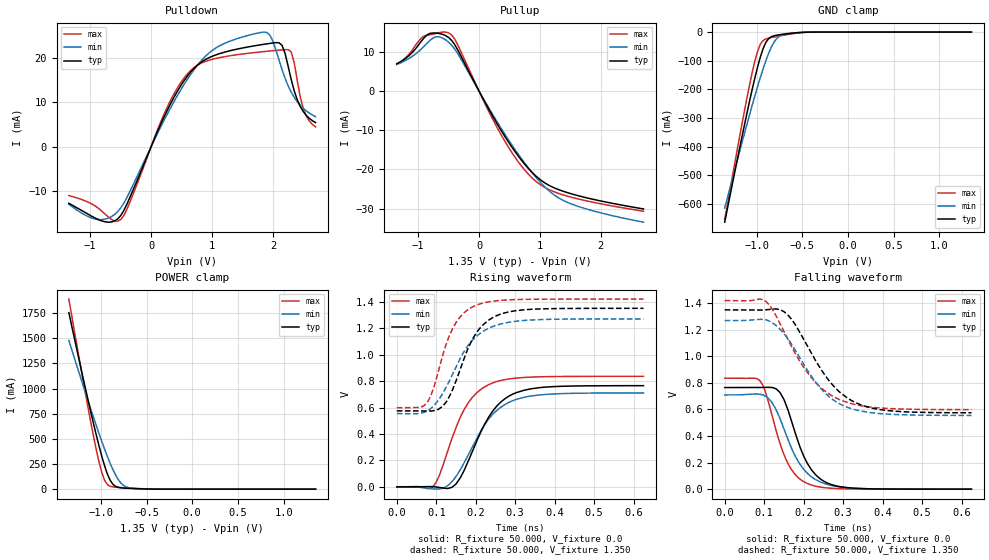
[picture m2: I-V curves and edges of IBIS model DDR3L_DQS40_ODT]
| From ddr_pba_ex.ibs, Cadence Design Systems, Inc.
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|   Model DDR3L_DQS40_ODT
[Model]   DDR3L_DQS40_ODT
Model_type I/O
Polarity   Non-Inverting
Enable   Active-High
Vinl   =   0.624V
Vinh   =   0.727V
C_comp   1.684pF   1.658pF   1.703pF
C_comp_pullup   0.506pF   0.522pF   0.489pF
C_comp_pulldown 1.177pF   1.136pF   1.213pF
[Model Spec]
Vinh   0.727V   NA   NA
Vinl   0.624V   NA   NA
Vmeas   0.675V   NA   NA
[Add Submodel]
|  Submodel_name   Mode
DDR3L_DQS_ODT60   Non-Driving
[Temperature Range]   27.000   0.125k   -40.000
[Voltage Range]   1.350V   1.270V   1.420V
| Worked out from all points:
|   slope of the pulldown table from 0 to 0.203 V, typ, clamps not added: 31.7 ohm
|   slope of the pullup table from 0 to 0.203 V, typ, clamps not added: 35 ohm
|   GND clamp passes 1 mA (typ) near -0.50 V on its own axis
|   POWER clamp passes 1 mA (typ) near -0.46 V on its own axis
|   rising waveform, R_fixture 50.000, V_fixture 0.0: 20-80 % time 78.8ps typ, 86.4ps min, 71.6ps max; typ from 0 V to 0.765 V
|   rising waveform, R_fixture 50.000, V_fixture 1.350: 20-80 % time 68.6ps typ, 82.9ps min, 58.3ps max; typ from 0.575 V to 1.35 V
|   falling waveform, R_fixture 50.000, V_fixture 0.0: 20-80 % time 59.7ps typ, 67.6ps min, 55.4ps max; typ from 0.765 V to 0 V
|   falling waveform, R_fixture 50.000, V_fixture 1.350: 20-80 % time 104ps typ, 102ps min, 106ps max; typ from 1.35 V to 0.575 V
[Pulldown]
|Voltage   I(typ)   I(min)   I(max)
-1.35V    -12.71mA   -12.95mA   -11mA
-850mV    -16.48mA   -16.4mA    -14.01mA
-500mV    -15.51mA   -13.79mA   -16.4mA
200mV     6.324mA    5.595mA    6.939mA
500mV     14.01mA    13.08mA    14.69mA
900mV     19.68mA    20.46mA    19.24mA
1.35V     21.77mA    24.03mA    20.58mA
1.95V     23.25mA    25.11mA    21.53mA
2.15V     22.81mA    17.35mA    21.79mA
2.3V      15.11mA    12.27mA    21.33mA
2.5V      7.867mA    8.611mA    8.524mA
2.7V      5.436mA    6.755mA    4.464mA
[Pullup]
|Voltage   I(typ)   I(min)   I(max)
-1.35V    6.994mA    6.778mA    6.785mA
-1.1V     9.771mA    8.81mA     10.37mA
-850mV    14.35mA    12.26mA    14.25mA
-700mV    14.79mA    13.87mA    14.72mA
-500mV    13.68mA    12.48mA    14.85mA
-350mV    10.51mA    9.572mA    11.81mA
400mV     -10.97mA   -10.4mA    -12.15mA
650mV     -16.69mA   -16.24mA   -18.16mA
900mV     -21.19mA   -21.37mA   -22.58mA
1.2V      -24.45mA   -26.1mA    -25.49mA
1.45V     -25.91mA   -28.39mA   -26.8mA
2.7V      -30.07mA   -33.45mA   -30.65mA
[GND_clamp]
|Voltage   I(typ)   I(min)   I(max)
-1.35V    -663.5mA   -614.2mA   -654.4mA
-1.17V    -379.6mA   -396.8mA   -336.4mA
-1.05V    -201.2mA   -256.6mA   -142.3mA
-990mV    -121.8mA   -190.1mA   -66.76mA
-960mV    -87.12mA   -158.5mA   -42.47mA
-930mV    -58.01mA   -128.3mA   -29.57mA
-870mV    -23.03mA   -74.64mA   -21.11mA
-810mV    -12.75mA   -34.94mA   -17.06mA
-750mV    -9.219mA   -14.09mA   -13.42mA
-690mV    -6.687mA   -6.669mA   -9.983mA
-420mV    -175.8uA   -266.9uA   -234.9uA
1.35V     1.781nA    307.1nA    267.4pA
[POWER_clamp]
|Voltage   I(typ)   I(min)   I(max)
-1.35V    1.755A     1.479A     1.89A
-1.17V    1.006A     962.6mA    958.1mA
-1.05V    538.4mA    632.4mA    392.2mA
-990mV    328mA      475.7mA    167mA
-960mV    234.7mA    400.6mA    90.32mA
-930mV    154.2mA    328.7mA    47.17mA
-900mV    91.53mA    260.8mA    29.3mA
-870mV    50.28mA    198.1mA    22.68mA
-780mV    13.3mA     60.49mA    15.94mA
-720mV    9.309mA    21.57mA    12.7mA
-660mV    6.902mA    8.818mA    9.643mA
1.35V     -4.773nA   -193.5nA   -1nA
[Ramp]
| variable   typ   min   max
dV/dt_r 0.459/79.862p   0.426/87.109p   0.502/73.280p
dV/dt_f 0.465/0.106n   0.429/0.104n   0.493/0.108n
R_load = 50.000
| The next line is not an IBIS keyword
| [Initial Delay]   0.200ns   0.400ns   0.150ns
[Rising Waveform]
R_fixture= 50.000
V_fixture= 0.0
V_fixture_min= 0.0
V_fixture_max= 0.0
|time   V(typ)   V(min)   V(max)
0s        6.488uV    823.9uV    -14.21uV
92ps      1.282mV    -15.85mV   3.07mV
107ps     -3.761mV   -16.06mV   80.39mV
141ps     -883.8uV   43.86mV    376mV
160ps     63.79mV    125.2mV    520.2mV
179ps     180mV      229.5mV    626.7mV
233ps     528.4mV    514.1mV    773.3mV
272ps     662.3mV    619.2mV    809.9mV
331ps     736.1mV    682.6mV    828.7mV
625ps     765.1mV    710mV      835.9mV
[Rising Waveform]
R_fixture= 50.000
V_fixture= 1.350
V_fixture_min= 1.270
V_fixture_max= 1.420
|time   V(typ)   V(min)   V(max)
0s        574.7mV    554.4mV    598.5mV
55ps      574.7mV    554.1mV    600.6mV
77ps      573.4mV    574.5mV    639.2mV
92ps      575.2mV    607.5mV    735.4mV
116ps     609mV      704mV      990.9mV
150ps     799.9mV    906.5mV    1.243V
197ps     1.143V     1.125V     1.368V
234ps     1.263V     1.201V     1.4V
292ps     1.328V     1.248V     1.415V
625ps     1.35V      1.27V      1.42V
[Falling Waveform]
R_fixture= 50.000
V_fixture= 0.0
V_fixture_min= 0.0
V_fixture_max= 0.0
|time   V(typ)   V(min)   V(max)
0s        765.2mV    709.9mV    835.9mV
89ps      764.7mV    715mV      816.8mV
104ps     766.5mV    698.1mV    725.4mV
131ps     753.2mV    592.7mV    433.6mV
150ps     676.2mV    454.8mV    261.8mV
166ps     544.1mV    331.2mV    161.6mV
211ps     186.5mV    115.4mV    40.48mV
240ps     81.86mV    57.68mV    16.52mV
290ps     19.7mV     17.21mV    3.851mV
625ps     29.82uV    61.65uV    34.44uV
[Falling Waveform]
R_fixture= 50.000
V_fixture= 1.350
V_fixture_min= 1.270
V_fixture_max= 1.420
|time   V(typ)   V(min)   V(max)
0s        1.35V      1.27V      1.42V
98ps      1.349V     1.278V     1.426V
119ps     1.355V     1.257V     1.363V
150ps     1.337V     1.172V     1.188V
180ps     1.234V     1.04V      1.015V
223ps     1.005V     835.7mV    827.6mV
293ps     726.9mV    639.6mV    671.3mV
339ps     641.7mV    592.2mV    631.8mV
389ps     601.2mV    570.1mV    612.5mV
625ps     575.1mV    555.3mV    598.8mV
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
